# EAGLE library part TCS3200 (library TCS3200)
High-Resolution Conversion of Light Intensity to Frequency Programmable Color and Full-Scale Output Frequency Communicates Directly With a Microcontroller Single-Supply Operation (2.7 V to 5.5 V) Power Down Feature Nonlinearity Error Typically 0.2% at 50 kHz Source: Datasheet
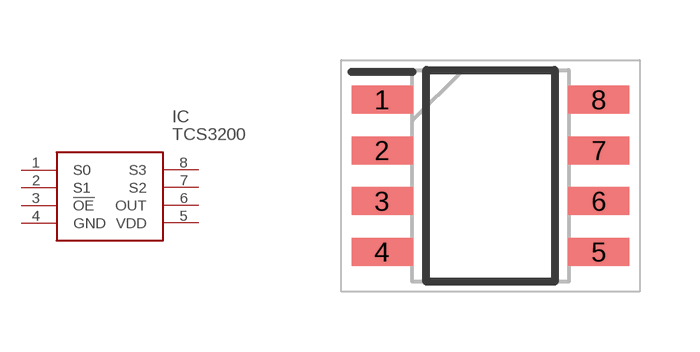
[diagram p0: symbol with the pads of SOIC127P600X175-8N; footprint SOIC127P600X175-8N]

Designator prefix IC

## TCS3200 (Description: High-Resolution Conversion of Light Intensity to Frequency Programmable Color and Full-Scale Output Frequency Communicates Directly With a Microcontroller Single-Supply Operation (2.7 V to 5.5 V) Power Down Feature Nonlinearity Error Typically 0.2% at 50 kHz; Height: 1.75mm; Manufacturer_Name: ams; Manufacturer_Part_Number: TCS3200; Mouser_Part_Number: N/A; Mouser_Price-Stock: https://www.mouser.co.uk/ProductDetail/ams/TCS3200?qs=N6LLV8I65%252BcsUeP7A1YMoQ%3D%3D)  [SOIC127P600X175-8N]
1  S0
2  S1
3  !OE
4  GND
5  VDD
6  OUT
7  S2
8  S3

## Footprint SOIC127P600X175-8N (pad centres in mm)
SOIC-8 - Package D_2021
smd 1.525 x 0.7: 1 -2.712,1.905; 2 -2.712,0.635; 3 -2.712,-0.635; 4 -2.712,-1.905; 5 2.712,-1.905; 6 2.712,-0.635; 7 2.712,0.635; 8 2.712,1.905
